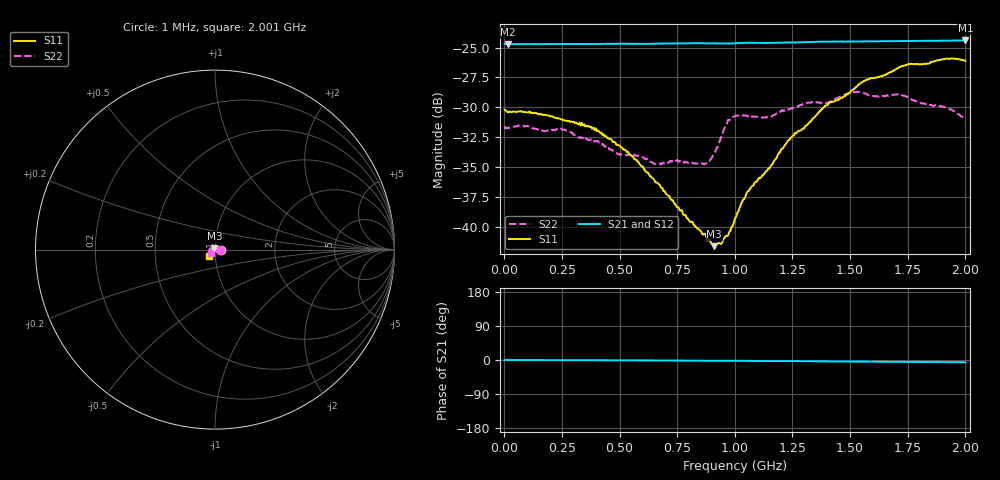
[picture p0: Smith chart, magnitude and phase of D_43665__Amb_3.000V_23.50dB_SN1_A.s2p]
! device id: 43665_
! dir: \\malibu\benchdata\1_engineers\tn_data\43665_75ohm\new\sparar\43665_\amb\3p000v\23p50db
! Serial: 1
! Insertion: A
! Temp: Amb
! VDD: 3.000V
! Attenuation Step: 23.50dB
! IDD: 1.448721e+00mA
! FILE NAME
! DATE 03-27-2009 08:39:08
! CORRECTED  DATA
#  Hz  S  RI  R  75
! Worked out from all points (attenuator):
!   401 points, 1 MHz to 2.001 GHz, reference 75 ohm
!   highest |S21| = -24.41 dB at 2.001 GHz (marker M1); lowest = -24.7 dB at 16 MHz (marker M2)
!   lowest |S11| = -41.6 dB at 911 MHz (marker M3), VSWR 1.02, Z = 74.4 + j1.1 ohm
!   |S11| at or under -10 dB: start of sweep to end of sweep
!   |S22| runs from -34.8 to -28.7 dB; largest |S21 - S12| = 0.0003
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1000000  0.0309 -0.000245  0.0583 -0.000117  0.0582 -1.53e-06  0.0263 -9.88e-06
1.6e7  0.0301 0.000344  0.058 -4.96e-05  0.0581 -6.86e-05  0.0258 0.000566
2.41e8  0.0277 0.00604  0.0581 -0.000348  0.0582 -0.000345  0.0225 0.0126
3.36e8  0.026 0.00803  0.0582 -0.000557  0.0582 -0.000536  0.0172 0.016
5.31e8  0.0175 0.0108  0.0583 -0.00101  0.0583 -0.001  0.00638 0.0188
6.71e8  0.0103 0.011  0.0584 -0.00124  0.0584 -0.00117  -0.0027 0.0181
7.41e8  0.00662 0.0105  0.0585 -0.00147  0.0585 -0.00137  -0.00725 0.0175
8.71e8  -0.00115 0.00928  0.0586 -0.00208  0.0586 -0.00191  -0.0155 0.00984
9.11e8  -0.00367 0.00742  0.0585 -0.00223  0.0585 -0.00209  -0.019 0.00698
9.61e8  -0.00631 0.00659  0.0583 -0.00217  0.0584 -0.00203  -0.0257 0.00633
1.001e9  -0.00895 0.00608  0.0585 -0.00211  0.0586 -0.00194  -0.028 0.00797
1.061e9  -0.0134 0.00432  0.0588 -0.00243  0.0589 -0.00227  -0.0287 0.00523
1.146e9  -0.0175 0.000976  0.0587 -0.00276  0.0588 -0.00261  -0.0288 0.00141
1.241e9  -0.0231 -0.00334  0.059 -0.00301  0.0591 -0.00287  -0.0308 -0.00428
1.336e9  -0.0271 -0.00781  0.0593 -0.00334  0.0594 -0.0032  -0.0322 -0.00862
1.406e9  -0.0303 -0.0122  0.0594 -0.00383  0.0596 -0.00365  -0.0304 -0.0132
1.501e9  -0.0328 -0.0162  0.0594 -0.00427  0.0595 -0.00415  -0.0325 -0.0164
1.561e9  -0.0351 -0.0205  0.0595 -0.00449  0.0597 -0.00443  -0.031 -0.0187
1.671e9  -0.0362 -0.0253  0.0596 -0.00501  0.0597 -0.00493  -0.0294 -0.0198
1.756e9  -0.0366 -0.031  0.0597 -0.00532  0.0598 -0.00532  -0.0266 -0.0221
1.921e9  -0.0352 -0.0363  0.0598 -0.00596  0.06 -0.00589  -0.023 -0.0213
2.001e9  -0.0325 -0.0374  0.0599 -0.00627  0.0599 -0.00636  -0.0197 -0.0199
